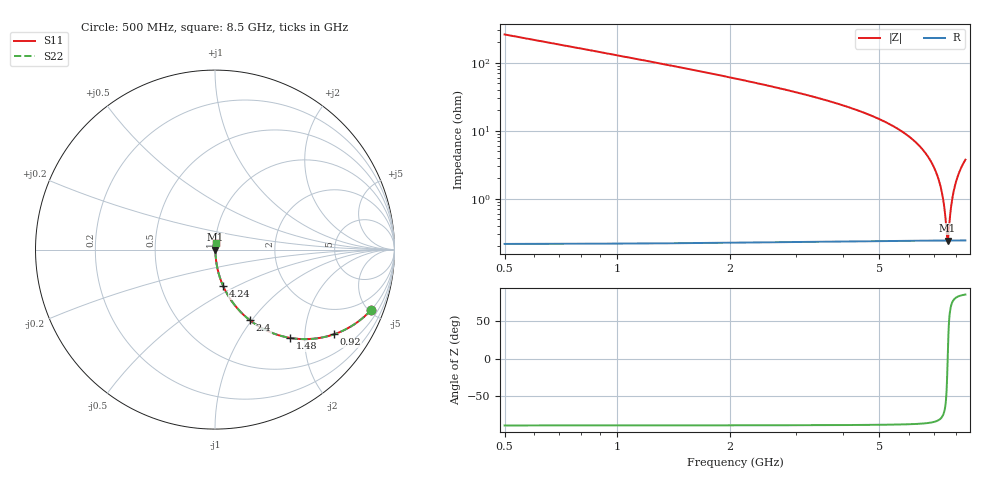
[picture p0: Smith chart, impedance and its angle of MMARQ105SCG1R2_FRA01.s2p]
! MMARQ105SCG1R2_FRA01  S-PARAMETER MODEL  ( General Type )
! Model Generated by TAIYO YUDEN Corporation (http://www.ty-top.com)
! Version 1.0
! TAIYO YUDEN Control No. 200326
! Copyright(c) 2020 TAIYO YUDEN CO.,LTD. All Rights Reserved.
! Product Description (link to TY-COMPAS)
! https://ds.yuden.co.jp/TYCOMPAS/or/detail?pn=MMARQ105SCG1R2BFRA01&u=M
! Products Name : Multilayer Ceramic Capacitors
! Characteristics :
!  Capacitance : 1.2 pF , Rated Voltage : 250V , TCC : CG / C0G
!  Case Size : 1.0 x 0.5 / 0.039 x 0.02 [mm/inch] , Thickness : 0.5 / 0.02 [mm/inch]
!  (Conditions: Temperature = 25 degC , DC Bias Current/Voltage = 0A / 0V)
! External Node Assignments :
!  1  o---| |---o  2
! GND o---------o GND
! Frequency Range : 500MHz  -  8.5GHz  [ 401 STEP ]
# MHz S RI R 50
! Freq[MHz].  S11 Real  S11 Imag  S21 Real  S21 Imag  S12 Real  S12 Imag  S22 Real  S22 Imag
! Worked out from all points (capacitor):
!   401 points, 500 MHz to 8.5 GHz, reference 50 ohm
!   read as one part in series: C = 1.22 pF near 540 MHz
!   lowest |Z| = 244 mohm at 7.62 GHz (marker M1)
!   series resonance near 7.622 GHz, so ESL is about 360 pH
!   S11 on the Smith chart (normalised r, x): 500 MHz: 1.00, -5.21; 920 MHz: 1.00, -2.80; 1.48 GHz: 1.00, -1.70; 2.4 GHz: 1.00, -0.98; 4.24 GHz: 1.00, -0.43; 8.5 GHz: 1.00, +0.07
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500  0.8714 -0.3343  0.1286 0.3343  0.1286 0.3343  0.8714 -0.3343
920  0.6624 -0.4721  0.3376 0.4721  0.3376 0.4721  0.6624 -0.4721
1480  0.42 -0.4923  0.58 0.4923  0.58 0.4923  0.42 -0.4923
1840  0.3101 -0.4609  0.6899 0.4609  0.6899 0.4609  0.3101 -0.4609
2400  0.1954 -0.3942  0.8046 0.3942  0.8046 0.3942  0.1954 -0.3942
3180  0.1051 -0.3033  0.8949 0.3033  0.8949 0.3033  0.1051 -0.3033
4240  0.0455 -0.2028  0.9545 0.2028  0.9545 0.2028  0.0455 -0.2028
4500  0.0367 -0.1819  0.9633 0.1819  0.9633 0.1819  0.0367 -0.1819
5840  0.0108 -0.0913  0.9892 0.0913  0.9892 0.0913  0.0108 -0.0913
6660  0.00456 -0.0461  0.9954 0.0461  0.9954 0.0461  0.00456 -0.0461
6960  0.00339 -0.031  0.9966 0.031  0.9966 0.031  0.00339 -0.031
7180  0.00284 -0.0204  0.9972 0.0204  0.9972 0.0204  0.00284 -0.0204
7320  0.00262 -0.0138  0.9974 0.0138  0.9974 0.0138  0.00262 -0.0138
7420  0.00251 -0.00918  0.9975 0.00918  0.9975 0.00918  0.00251 -0.00918
7500  0.00246 -0.00552  0.9975 0.00552  0.9975 0.00552  0.00246 -0.00552
7580  0.00243 -0.00189  0.9976 0.00189  0.9976 0.00189  0.00243 -0.00189
7620  0.00243 -9.48e-05  0.9976 9.48e-05  0.9976 9.48e-05  0.00243 -9.48e-05
7660  0.00243 0.00169  0.9976 -0.00169  0.9976 -0.00169  0.00243 0.00169
7800  0.00249 0.00788  0.9975 -0.00788  0.9975 -0.00788  0.00249 0.00788
7940  0.00263 0.014  0.9974 -0.014  0.9974 -0.014  0.00263 0.014
8180  0.00302 0.0241  0.997 -0.0241  0.997 -0.0241  0.00302 0.0241
8500  0.00383 0.0372  0.9962 -0.0372  0.9962 -0.0372  0.00383 0.0372
